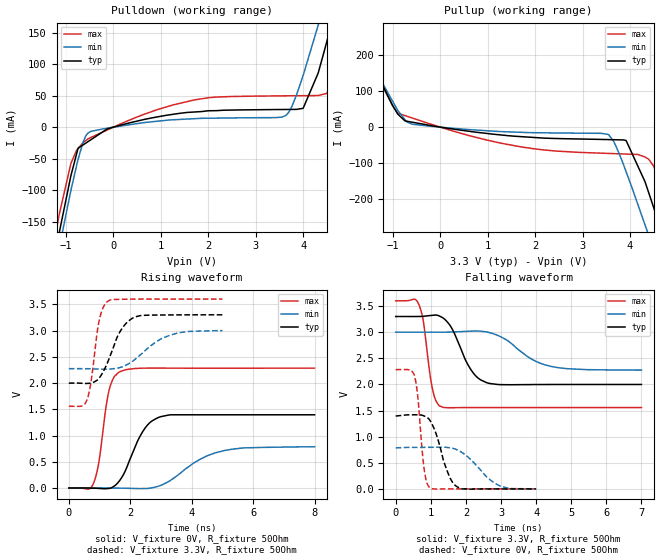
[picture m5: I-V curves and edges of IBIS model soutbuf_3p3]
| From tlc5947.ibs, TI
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|   soutbuf_3p3 Model
[Model]   soutbuf_3p3
Model_type   Output
Polarity   Non-Inverting
Vmeas = 1.65
Vref = 1.65
Cref = 15pF
Rref = 50
|   typ   min   max
|   (nom PVT)   (Fast PVT)   (slow PVT)
|Average
C_comp   3.523e-12   3.460e-12   3.712e-12
|ON state : BUFFER OUTPUT TURNED HIGH
|C_comp   3.523e-12   3.460e-12   3.712e-12
|OFF state: BUFFER OUTPUT TURNED LOW
|C_comp   2.715e-12   2.526e-12   2.785e-12
| Where nom  PVT is Nominal Process,  3.3V,  65C
|   Fast PVT is Strong Process,   3.6V,  -40C
|   Slow PVT is Weak Process,   3V,  125C
[Voltage Range]   3.3   3   3.6
|Ambient Temperature   25   85   -40
|Junction Temperature
[Temperature Range]   65   125   -40
[Pullup Reference]   3.3   3   3.6
[Pulldown Reference]   0   0   0
[Power Clamp Reference]   3.3   3   3.6
[GND Clamp Reference]   0   0   0
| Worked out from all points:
|   slope of the pulldown table from 0 to 0.495 V, typ, clamps not added: 52.1 ohm
|   slope of the pullup table from 0 to 0.495 V, typ, clamps not added: 52 ohm
|   falling waveform, V_fixture 3.3V, R_fixture 50Ohm: 20-80 % time 541ps typ, 919ps min, 241ps max; typ from 3.3 V to 2 V
|   rising waveform, V_fixture 0V, R_fixture 50Ohm: 20-80 % time 653ps typ, 1.23ns min, 329ps max; typ from 0 V to 1.4 V
|   rising waveform, V_fixture 3.3V, R_fixture 50Ohm: 20-80 % time 576ps typ, 969ps min, 283ps max; typ from 2 V to 3.3 V
|   falling waveform, V_fixture 0V, R_fixture 50Ohm: 20-80 % time 388ps typ, 698ps min, 177ps max; typ from 1.4 V to 0 V
[Pulldown]
|   Voltage   I(typ)   I(min)   I(max)
-3.3V     -1.06A     -1.03A     -1.12A
-1.135V   -164.7mA   -188.5mA   -136mA
-745.8mV  -33.5mA    -51.44mA   -33.81mA
-474mV    -19.91mA   -6.706mA   -16.39mA
1.706V    24.03mA    13.42mA    43.18mA
3.636V    28.03mA    18.62mA    49.72mA
4V        29.86mA    82.23mA    49.94mA
4.314V    85.36mA    161mA      50.11mA
4.583V    160.6mA    232mA      71.66mA
4.723V    202.3mA    269.9mA    114.6mA
5.208V    346.6mA    400.9mA    280.6mA
6.6V      784.3mA    791.1mA    798.6mA
[Pullup]
|   Voltage   I(typ)   I(min)   I(max)
-3.3V     757.8mA    691.4mA    875.2mA
-1.789V   282.8mA    273.4mA    305.2mA
-1.692V   254.7mA    246.7mA    269.9mA
-1.004V   60.21mA    71.74mA    58.92mA
-591mV    13.73mA    8.273mA    25.29mA
1.706V    -26.46mA   -14.45mA   -55.05mA
3.54V     -34.64mA   -20.42mA   -73.12mA
3.917V    -37.21mA   -123.9mA   -74.89mA
4.392V    -181.8mA   -301.1mA   -89.19mA
4.662V    -291.1mA   -405.4mA   -171.8mA
4.986V    -424.3mA   -531.8mA   -315.7mA
6.6V      -1.099A    -1.168A    -1.062A
[Ramp]
R_load = 50
|   typ   min   max
dV/dt_r   0.850608/6.70069e-10   0.477032/1.25484e-09   1.37008/3.28832e-10
dV/dt_f   0.780553/5.40417e-10   0.435668/9.18718e-10   1.2255/2.40758e-10
[Falling Waveform]
V_fixture = 3.3V
V_fixture_min = 3V
V_fixture_max = 3.6V
R_fixture = 50Ohm
|   Time   V(typ)   V(min)   V(max)
0s        3.3V       3V         3.6V
675ps     3.301V     3V         3.505V
800ps     3.305V     3V         3.156V
1.05ns    3.323V     3V         1.906V
1.25ns    3.308V     3V         1.589V
1.575ns   3.101V     3.003V     1.555V
2.2ns     2.228V     3.022V     1.557V
2.6ns     2.032V     3.003V     1.558V
4.425ns   1.999V     2.345V     1.558V
7ns       1.999V     2.274V     1.557V
[Rising Waveform]
V_fixture = 0V
V_fixture_min = 0V
V_fixture_max = 0V
R_fixture = 50Ohm
|   Time   V(typ)   V(min)   V(max)
0s        402.4pV    3.14nV     326.4pV
800ps     -2.764mV   398.6uV    85.26mV
975ps     -7.462mV   448.4uV    480.4mV
1.3ns     -8.26mV    -254uV     1.837V
1.45ns    25.47mV    -1.024mV   2.091V
1.65ns    138.1mV    -2.463mV   2.212V
2.4ns     1.069V     -10.52mV   2.283V
2.925ns   1.346V     36.09mV    2.285V
5.025ns   1.395V     709.1mV    2.283V
8ns       1.395V     786mV      2.283V
[Rising Waveform]
V_fixture = 3.3V
V_fixture_min = 3V
V_fixture_max = 3.6V
R_fixture = 50Ohm
|   Time   V(typ)   V(min)   V(max)
0s        1.999V     2.274V     1.557V
450ps     1.995V     2.274V     1.568V
600ps     1.993V     2.273V     1.693V
725ps     1.998V     2.271V     2.034V
975ps     2.086V     2.266V     3.151V
1.25ns    2.376V     2.265V     3.55V
1.675ns   2.987V     2.297V     3.595V
2.125ns   3.251V     2.437V     3.599V
3.325ns   3.298V     2.916V     3.6V
5ns       3.3V       3V         3.6V
[Falling Waveform]
V_fixture = 0V
V_fixture_min = 0V
V_fixture_max = 0V
R_fixture = 50Ohm
|   Time   V(typ)   V(min)   V(max)
0s        1.395V     786mV      2.284V
525ps     1.419V     794.8mV    2.189V
625ps     1.418V     794.9mV    1.797V
800ps     1.399V     795.5mV    433.6mV
950ps     1.335V     796.5mV    36.71mV
1.15ns    1.056V     798.3mV    -2.276mV
1.5ns     287mV      790.9mV    309uV
1.725ns   51.62mV    755.2mV    283.1uV
2.925ns   183.2uV    72.04mV    295uV
4ns       115.8uV    364.3uV    202uV
